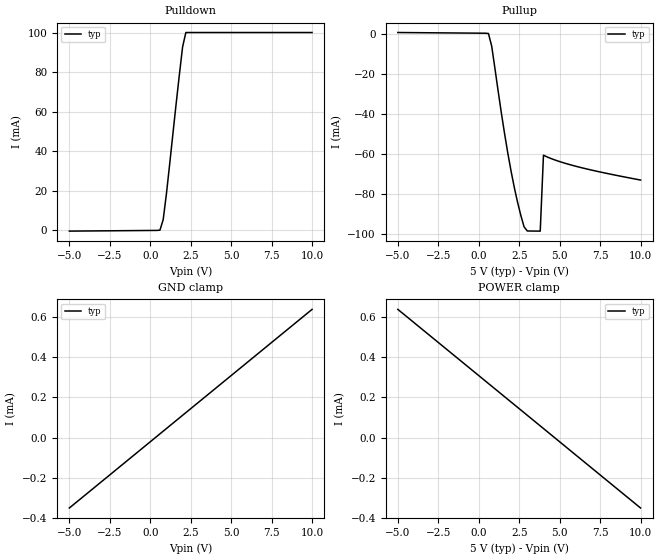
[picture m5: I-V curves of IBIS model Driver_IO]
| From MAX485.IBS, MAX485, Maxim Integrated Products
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|   Driver Input/Output A & B
[Model]   Driver_IO
|Signals   A, B
Model_type   I/O
Vinl = 0.8V
Vinh = 2.0V
C_comp   0.538pF   NA   NA
[Temperature Range]   25   -40   85
[Voltage Range]   5.00V   4.75V   5.25V
[Pullup Reference]   5.00V   4.75V   5.25V
[Pulldown Reference]   0.00V   0.00V   0.00V
[POWER Clamp Reference]   5.00V   4.75V   5.25V
[GND Clamp Reference]   0.00V   0.00V   0.00V
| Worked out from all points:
|   slope of the pulldown table from 0 to 0.75 V, typ, clamps not added: 181 ohm
|   slope of the pullup table from 0 to 0.75 V, typ, clamps not added: 154 ohm
[Pullup]
| Note that the[Pullup]voltage table is referenced to Vcc
| and is calculated using Vtable=Vcc - Vmeasured.
| V(V)  I(typ)   I(min)  I(max)
-5V       638.4uA    NA         NA
600mV     143uA      NA         NA
800mV     -6.145mA   NA         NA
1.4V      -39.74mA   NA         NA
2V        -68.78mA   NA         NA
2.6V      -90.78mA   NA         NA
2.8V      -96.5mA    NA         NA
3V        -98.61mA   NA         NA
3.8V      -98.68mA   NA         NA
4V        -60.72mA   NA         NA
6V        -66.24mA   NA         NA
10V       -73.15mA   NA         NA
[Pulldown]
| Note that the[Pulldown]voltage table is referenced to Gnd.
| Also, the Semiconductor Parameter Analyzer (Force and Sense)
| clamps the supply current to 100mA to protect the system.
| V(V)  I(typ)   I(min)  I(max)
-5V       -351.2uA   NA         NA
600mV     131.6uA    NA         NA
800mV     5.457mA    NA         NA
1V        18.47mA    NA         NA
1.6V      63.98mA    NA         NA
1.8V      78.67mA    NA         NA
2V        92.74mA    NA         NA
2.2V      100mA      NA         NA
10V       100mA      NA         NA
[POWER_clamp]
| Note that the[POWER_clamp]voltage table is referenced to Vcc
| and is calculated using Vtable=Vcc - Vmeasured.
| V(V)  I(typ)   I(min)  I(max)
-5V       638.7uA    NA         NA
400mV     282.5uA    NA         NA
6V        -87.28uA   NA         NA
10V       -351.2uA   NA         NA
[GND_clamp]
| Note that the[GND_clamp]voltage table is referenced to Gnd.
| V(V)  I(typ)   I(min)  I(max)
-5V       -351.2uA   NA         NA
-1V       -87.28uA   NA         NA
4.6V      282.5uA    NA         NA
10V       638.8uA    NA         NA
[Ramp]
| variable   typ   min   max
dV/dt_r   2.67/23nS   NA   NA
dV/dt_f   2.40/11nS   NA   NA
R_load = 5Kohms
|End [Model] Driver_IO
|End [Component] MAX485
